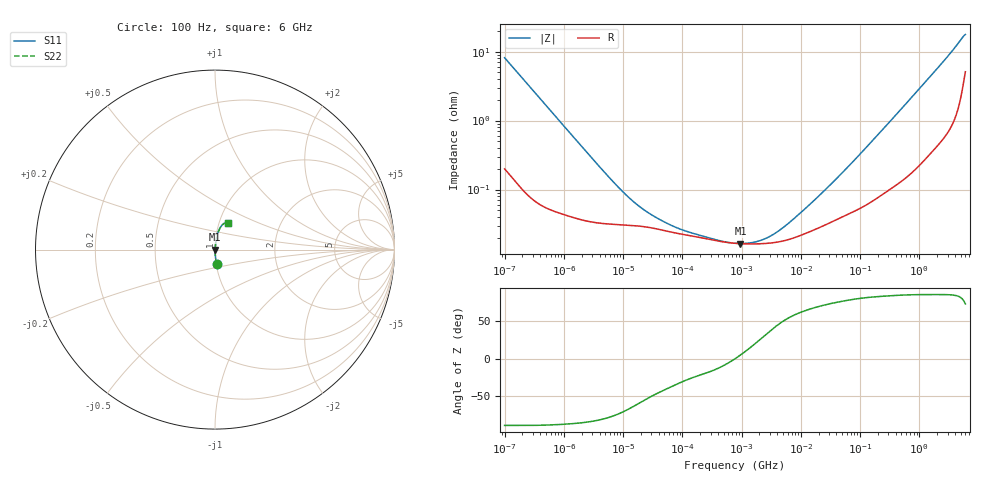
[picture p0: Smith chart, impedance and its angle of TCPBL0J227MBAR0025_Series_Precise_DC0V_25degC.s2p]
! TCPBL0J227MBAR0025 Polymer Tantalum Capacitor Sparameter Model
! Model Generated by Samsung Electro-Mechanics
! Samsung Sparameter Version 5.0
! Date : Oct-21-2025
! Products : Polymer Tantalum Capacitor
! Characteristics :
!  Nominal Capacitance = 220uF
!  Capacitance Tolerance = +/-20%
!  ESR = 25 mohm max at 100kHz
!  Rated Voltage = 6.3Vdc
!  Size = 1411(unit:inch), 3528(unit:mm)
!  Length = 3.50+/-0.20mm
!  Width = 2.80+/-0.20mm
!  Thickness = 1.90+/-0.10mm
!  Lineup = Conductive Polymer Type
!  Feature = PBL
!  Measurement Temperature : 25degC.
!  DC bias Value = 0V
!  Frequency : 100Hz ~ 6GHz
! External Node Assignments :
!  1  o---||---o  2
# MHz S RI R 50.0
! Freq.  Real(S11)  Im(S11)  Real(S12)  Im(S12)  Real(S21)  Im(S21)  Real(S22)  Im(S22)
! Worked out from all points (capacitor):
!   300 points, 100 Hz to 6 GHz, reference 50 ohm
!   read as one part in series: C = 195 uF near 106.2 Hz
!   lowest |Z| = 16.5 mohm at 955.3 kHz (marker M1)
!   series resonance near 768.6 kHz, so ESL is about 220 pH
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0.0001  0.00854 -0.0806  0.9915 0.0806  0.9915 0.0806  0.00854 -0.0806
0.0003120785  0.00139 -0.0264  0.9986 0.0264  0.9986 0.0264  0.00139 -0.0264
0.001998454  0.000381 -0.00421  0.9996 0.00421  0.9996 0.00421  0.000381 -0.00421
0.006236745  0.000317 -0.00137  0.9997 0.00137  0.9997 0.00137  0.000317 -0.00137
0.01205343  0.000305 -0.000728  0.9997 0.000728  0.9997 0.000728  0.000305 -0.000728
0.02066501  0.000293 -0.000449  0.9997 0.000449  0.9997 0.000449  0.000293 -0.000449
0.03993819  0.000265 -0.000265  0.9997 0.000265  0.9997 0.000265  0.000265 -0.000265
0.0726988  0.000237 -0.000168  0.9998 0.000168  0.9998 0.000168  0.000237 -0.000168
0.1246385  0.000217 -0.000112  0.9998 0.000112  0.9998 0.000112  0.000217 -0.000112
0.4129808  0.000179 -3.82e-05  0.9998 3.82e-05  0.9998 3.82e-05  0.000179 -3.82e-05
0.7981464  0.000166 2.51e-06  0.9998 -2.51e-06  0.9998 -2.51e-06  0.000166 2.51e-06
0.9552658  0.000165 1.47e-05  0.9998 -1.47e-05  0.9998 -1.47e-05  0.000165 1.47e-05
1.738854  0.000163 6.28e-05  0.9998 -6.28e-05  0.9998 -6.28e-05  0.000163 6.28e-05
3.165205  0.000168 0.000134  0.9998 -0.000134  0.9998 -0.000134  0.000168 0.000134
5.761569  0.000185 0.000247  0.9998 -0.000247  0.9998 -0.000247  0.000185 0.000247
15.95059  0.000256 0.000618  0.9997 -0.000618  0.9997 -0.000618  0.000256 0.000618
63.25518  0.000445 0.00211  0.9996 -0.00211  0.9996 -0.00211  0.000445 0.00211
318.7652  0.00109 0.0096  0.9989 -0.0096  0.9989 -0.0096  0.00109 0.0096
1190.629  0.00376 0.0339  0.9962 -0.0339  0.9962 -0.0339  0.00376 0.0339
3104.549  0.0143 0.0857  0.9857 -0.0857  0.9857 -0.0857  0.0143 0.0857
4721.671  0.0345 0.1305  0.9655 -0.1305  0.9655 -0.1305  0.0345 0.1305
6000  0.0727 0.1497  0.9273 -0.1497  0.9273 -0.1497  0.0727 0.1497
